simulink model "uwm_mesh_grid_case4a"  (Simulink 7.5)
settings: Solver=ode45  StartTime=0.0  StopTime=3.0  RelTol=1e-4
undefined symbols (not defined in the file or in its folder): D1, Delta, dfilt, DiscIntNeverNeededParam
libraries: powerlib x86, powerlib_extras x20, dsparch4 x6
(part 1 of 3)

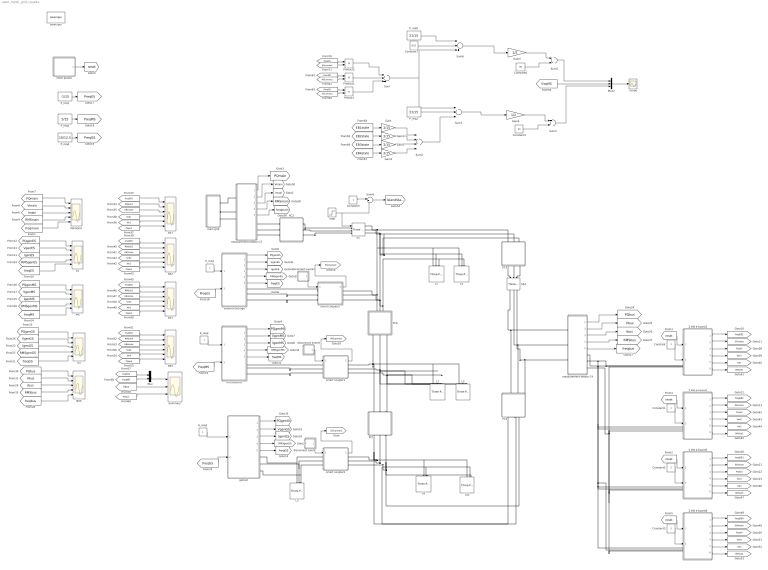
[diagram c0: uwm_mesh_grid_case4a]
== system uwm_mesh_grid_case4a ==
  2 kW e-board1 : Subsystem
  2 kW e-board2 : Subsystem
  2 kW e-board3 : Subsystem
  2 kW e-board4 : Subsystem
  BUS : Scope  NumInputPorts=5
  Constant{,1..3} (4 alike) : Constant  Value=2  OutDataType=fixdt(1, 16)  OutScaling=2^0
  Constant4 : Constant  Value=60  OutDataType=fixdt(1, 16)  OutScaling=2^0
  Constant5 : Constant  OutDataType=fixdt(1, 16)  OutScaling=2^0
  Constant6 : Constant  Value=60  OutDataType=fixdt(1, 16)  OutScaling=2^0
  Constant7 : Constant  Value=8/15  OutDataType=fixdt(1, 16)  OutScaling=2^0
  EB{1..4} (4 alike) : Scope  NumInputPorts=6
  ES : Scope  NumInputPorts=5
  E_req1 : Constant  OutDataType=fixdt(1, 16)  OutScaling=2^0
  E_req2 : Constant  OutDataType=fixdt(1, 16)  OutScaling=2^0
  E_req3 : Constant  OutDataType=fixdt(1, 16)  OutScaling=2^0
  GS : Scope  NumInputPorts=5
  Gain{,1..3} (4 alike) : Gain  Gain=2/15  ParameterDataType=fixdt(1, 16)  ParameterScaling=2^0  OutDataType=fixdt(1, 16)  OutScaling=2^0
  Gain4 : Gain  Gain=1/2  ParameterDataType=fixdt(1, 16)  ParameterScaling=2^0  OutDataType=fixdt(1, 16)  OutScaling=2^0
  Gain5 : Gain  Gain=1/2  ParameterDataType=fixdt(1, 16)  ParameterScaling=2^0  OutDataType=fixdt(1, 16)  OutScaling=2^0
  L{1..4,42} (5 alike) : powerlib/Elements/Three-Phase Series RLC Load  DialogController=POWERSYS.PowerSysDialog  PhysicalDomain=powersysdomain  SubClassName=unknown  LeftPortType=p1  RightPortType=p1  LConnTagsString=A|B|C  Configuration=Y (grounded)  NominalVoltage=208  NominalFrequency=60  ActivePower=4000  InductivePower=0  CapacitivePower=0  Measurements=None
  L5 : powerlib/Elements/Three-Phase Series RLC Load  DialogController=POWERSYS.PowerSysDialog  PhysicalDomain=powersysdomain  SubClassName=unknown  LeftPortType=p1  RightPortType=p1  LConnTagsString=A|B|C  Configuration=Y (grounded)  NominalVoltage=208  NominalFrequency=60  ActivePower=2000  InductivePower=0  CapacitivePower=0  Measurements=None
  L6 : powerlib/Elements/Three-Phase Series RLC Load  DialogController=POWERSYS.PowerSysDialog  PhysicalDomain=powersysdomain  SubClassName=unknown  LeftPortType=p1  RightPortType=p1  LConnTagsString=A|B|C  Configuration=Y (grounded)  NominalVoltage=208  NominalFrequency=60  ActivePower=2000  InductivePower=0  CapacitivePower=0  Measurements=None
  MS : Scope  NumInputPorts=5
  MainGrid : Scope  NumInputPorts=5
  Mux : Mux  Inputs=2
  Mux2 : Mux  Inputs=3
  PC2 : Subsystem  mask{R=.002810, L=.000679, C=2894.3}
  PC3 : Subsystem  mask{R=0.027352, L=.006600, C=288.6}
  PC4 : Subsystem  mask{R=.01688, L=.004070, C=336.7}
  PC5 : Subsystem  mask{R=.002600, L=.000640, C=2020.1}
  PC6 : Subsystem  mask{R=.013700, L=.003300, C=577.2}
  P_req1 : Constant  Value=-1/15  OutDataType=fixdt(1, 16)  OutScaling=2^0
  P_req2 : Constant  Value=21/15  OutDataType=fixdt(1, 16)  OutScaling=2^0
  P_req3 : Constant  Value=5/15  OutDataType=fixdt(1, 16)  OutScaling=2^0
  P_req4 : Constant  Value=10/12.5  OutDataType=fixdt(1, 16)  OutScaling=2^0
  P_req5 : Constant  Value=21/15  OutDataType=fixdt(1, 16)  OutScaling=2^0
  Product : Product  OutDataType=fixdt(1, 16)  OutScaling=2^0
  Product1 : Product  OutDataType=fixdt(1, 16)  OutScaling=2^0
  Product2 : Product  OutDataType=fixdt(1, 16)  OutScaling=2^0
  SS : powerlib/Elements/Three-Phase Breaker  DialogController=POWERSYS.PowerSysDialog  SystemSampleTime=-1  InitialState=closed  SwitchA=on  SwitchB=on  SwitchC=on  SwitchTimes=[1.]  External=on  BreakerResistance=.001  SnubberResistance=1e6  SnubberCapacitance=inf  Measurements=None
  SS3 : powerlib/Elements/Three-Phase Breaker  DialogController=POWERSYS.PowerSysDialog  SystemSampleTime=-1  InitialState=closed  SwitchA=on  SwitchB=on  SwitchC=on  SwitchTimes=[50]  External=off  BreakerResistance=.00001  SnubberResistance=1e10  SnubberCapacitance=inf  Measurements=None
  Scope : Scope
  Step : Step  Time=.5  Before=1  After=0  SampleTime=0
  Sum : Sum  Inputs=+++  OutDataType=fixdt(1, 16)  OutScaling=2^0
  Sum1 : Sum  Inputs=+--  OutDataType=fixdt(1, 16)  OutScaling=2^0
  Sum2 : Sum  Inputs=++++  OutDataType=fixdt(1, 16)  OutScaling=2^0
  Sum3 : Sum  OutDataType=fixdt(1, 16)  OutScaling=2^0
  Sum4 : Sum  Inputs=|+-  OutDataType=fixdt(1, 16)  OutScaling=2^0
  Sum5 : Sum  OutDataType=fixdt(1, 16)  OutScaling=2^0
  Sum6 : Sum  Inputs=--+  OutDataType=fixdt(1, 16)  OutScaling=2^0
  Summary : Scope  NumInputPorts=3
  disconnect event : Subsystem  mask{tstart=50, tstop=60}
      mask prompts: tstart "disconnect time"; tstop "connect time"
  disconnect event1 : Subsystem  mask{tstart=1, tstop=1.5}
      mask prompts: tstart "disconnect time"; tstop "connect time"
  disconnect event2 : Subsystem  mask{tstart=50, tstop=60}
      mask prompts: tstart "disconnect time"; tstop "connect time"
  external storage : Subsystem  AncestorBlock=|
      | UWM_blocks/inverter-based
      | DG (simplified)
      | 208V - 15kVA
  genset : Subsystem
  main grid : Subsystem
  measurement feeder C3 : Subsystem
  measurement feeder C4 : Subsystem
  microsource : Subsystem  AncestorBlock=|
      | UWM_blocks/inverter-based
      | DG (simplified)
      | 208V - 15kVA
  powergui : powerlib/powergui  Priority=1  SystemSampleTime=-1  SimulationMode=Discrete  SampleTime=20e-6  frequency=60  SPID=off  DisableSnubberDevices=off  DisableRonSwitches=off  DisableVfSwitches=off  SwTol=0  Interpol=off  frequencyindice=60  echomessages=off  HookPort=off  DisplayEquations=off  FunctionMessages=off  EnableUseOfTLC=off  x0status=steady  RestoreLinks=no  ResistiveCurrentMeasurement=off  Frange=[0:2:500]  Ylog=off  Xlog=on  ShowGrid=off  save=off  variable=ZData  ZoomFFT=on  StartTime=0.0  cycles=1  DisplayStyle=1  fundamental=60  FreqAxis=off  MaxFrequency=1000  frequencyindicesteady=1  RmsSteady=2  display=off  Ts=0  methode=off
  reset pulses : Subsystem  mask{tpulse=[50 100]}
  smart coupler1 : Subsystem
  smart coupler2 : Subsystem
  smart coupler3 : Subsystem
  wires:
  [PreqMS] -> microsource/2(P_req)
  E_req2/1 -> microsource/1(E_req)
  E_req1/1 -> external storage/1(E_req)
  E_req3/1 -> genset/1(Ereq)
  [PreqGS] -> genset/2(Preq)
  reset pulses/1(Out1) -> [reset]
  [reset] -> 2 kW e-board1/1(reset)
  2 kW e-board1/1(w) -> [freqEB1]
  2 kW e-board1/2(state) -> [EB1state]
  measurement feeder C3/3(I) -> [Imain]
  measurement feeder C3/1(PQ) -> [PQmain]
  [PreqES] -> external storage/2(P_req)
  P_req1/1 -> [PreqES]
  P_req3/1 -> [PreqMS]
  P_req4/1 -> [PreqGS]
  measurement feeder C3/2(V) -> [Vmain]
  [PQmain] -> MainGrid/1
  [Vmain] -> MainGrid/2
  [Imain] -> MainGrid/3
  [RMSmain] -> MainGrid/4
  external storage/5(freq) -> [freqES]
  external storage/3(I) -> [IgenES]
  external storage/2(V) -> [VgenES]
  external storage/1(PQ) -> [PQgenES]
  microsource/1(PQ) -> [PQgenMS]
  microsource/2(V) -> [VgenMS]
  microsource/3(I) -> [IgenMS]
  microsource/5(freq) -> [freqMS]
  genset/1(PQ) -> [PQgenGS]
  genset/2(V) -> [VgenGS]
  genset/3(I) -> [IgenGS]
  genset/5(freq) -> [freqGS]
  measurement feeder C4/1(PQ) -> [PQbus]
  measurement feeder C4/2(V) -> [Vbus]
  measurement feeder C4/3(I) -> [Ibus]
  measurement feeder C4/5(freq) -> [freqbus]
  measurement feeder C3/4(RMS) -> [RMSmain]
  external storage/4(RMS) -> [RMSgenES]
  microsource/4(RMS) -> [RMSgenMS]
  genset/4(RMS) -> [RMSgenGS]
  measurement feeder C3/5(freq) -> [freqmain]
  [freqmain] -> MainGrid/5
  [PQgenES] -> ES/1
  [VgenES] -> ES/2
  [IgenES] -> ES/3
  [RMSgenES] -> ES/4
  [freqES] -> ES/5
  [PQgenMS] -> MS/1
  [VgenMS] -> MS/2
  [IgenMS] -> MS/3
  [RMSgenMS] -> MS/4
  [freqMS] -> MS/5
  [PQgenGS] -> GS/1
  [VgenGS] -> GS/2
  [IgenGS] -> GS/3
  [RMSgenGS] -> GS/4
  [freqGS] -> GS/5
  measurement feeder C4/4(RMS) -> [RMSbus]
  [PQbus] -> BUS/1
  [Vbus] -> BUS/2
  [Ibus] -> BUS/3
  [RMSbus] -> BUS/4
  [freqbus] -> BUS/5
  Constant/1 -> 2 kW e-board1/2(priority)
  [freqEB1] -> EB1/1
  [RMSeb1] -> EB1/2
  [EB1state] -> EB1/3
  2 kW e-board1/3(PQ) -> [PQeb1]
  2 kW e-board1/4(V) -> [Veb1]
  2 kW e-board1/5(I) -> [Ieb1]
  2 kW e-board1/6(RMS) -> [RMSeb1]
  [PQeb1] -> EB1/6
  [Ieb1] -> EB1/5
  [Veb1] -> EB1/4
  [reset] -> 2 kW e-board2/1(reset)
  2 kW e-board2/1(w) -> [freqEB2]
  2 kW e-board2/2(state) -> [EB2state]
  Constant1/1 -> 2 kW e-board2/2(priority)
  2 kW e-board2/3(PQ) -> [PQeb2]
  2 kW e-board2/4(V) -> [Veb2]
  2 kW e-board2/5(I) -> [Ieb2]
  2 kW e-board2/6(RMS) -> [RMSeb2]
  [reset] -> 2 kW e-board3/1(reset)
  2 kW e-board3/1(w) -> [freqEB3]
  2 kW e-board3/2(state) -> [EB3state]
  Constant2/1 -> 2 kW e-board3/2(priority)
  2 kW e-board3/3(PQ) -> [PQeb3]
  2 kW e-board3/4(V) -> [Veb3]
  2 kW e-board3/5(I) -> [Ieb3]
  2 kW e-board3/6(RMS) -> [RMSeb3]
  [reset] -> 2 kW e-board4/1(reset)
  2 kW e-board4/1(w) -> [freqEB4]
  2 kW e-board4/2(state) -> [EB4state]
  Constant3/1 -> 2 kW e-board4/2(priority)
  2 kW e-board4/3(PQ) -> [PQeb4]
  2 kW e-board4/4(V) -> [Veb4]
  2 kW e-board4/5(I) -> [Ieb4]
  2 kW e-board4/6(RMS) -> [RMSeb4]
  [freqEB2] -> EB2/1
  [RMSeb2] -> EB2/2
  [EB2state] -> EB2/3
  [PQeb2] -> EB2/6
  [Ieb2] -> EB2/5
  [Veb2] -> EB2/4
  [freqEB3] -> EB3/1
  [RMSeb3] -> EB3/2
  [EB3state] -> EB3/3
  [PQeb3] -> EB3/6
  [Ieb3] -> EB3/5
  [Veb3] -> EB3/4
  [freqEB4] -> EB4/1
  [RMSeb4] -> EB4/2
  [EB4state] -> EB4/3
  [PQeb4] -> EB4/6
  [Ieb4] -> EB4/5
  [Veb4] -> EB4/4
  Step/1 -> SS/1, Sum4/2
  [freqEB4] -> Mux/1
  [freqMS] -> Mux/2
  [PQbus] -> Summary/3
  Mux/1 -> Summary/1
  [Vbus] -> Summary/2
  disconnect event/1(Out1) -> smart coupler2/1(event)
  Product2/1 -> Sum/1
  Product1/1 -> Sum/2
  smart coupler2/1(connected) -> [GSconnect]
  [PreqGS] -> Product/1
  [GSconnect] -> Product/2
  Product/1 -> Sum/3
  Constant5/1 -> Sum4/1
  Sum4/1 -> [IslandState]
  Constant6/1 -> Sum5/2
  Gain5/1 -> Sum5/1
  Sum6/1 -> Gain5/1
  [freqMS] -> Mux2/2
  Sum5/1 -> Mux2/1
  [EB1state] -> Gain/1
  P_req2/1 -> Sum1/2
  [EB2state] -> Gain1/1
  [EB3state] -> Gain2/1
  [EB4state] -> Gain3/1
  Gain1/1 -> Sum2/2
  Gain2/1 -> Sum2/3
  Gain/1 -> Sum2/1
  Gain3/1 -> Sum2/4
  Sum2/1 -> Sum1/3
  Constant4/1 -> Sum3/2
  Gain4/1 -> Sum3/1
  Sum1/1 -> Gain4/1
  Mux2/1 -> Scope/1
  Sum3/1 -> Mux2/3
  Sum/1 -> Sum1/1, Sum6/3
  Constant7/1 -> Sum6/2
  P_req5/1 -> Sum6/1
  disconnect event1/1(Out1) -> smart coupler1/1(event)
  smart coupler1/1(connected) -> [MSconnect]
  disconnect event2/1(Out1) -> smart coupler3/1(event)
  smart coupler3/1(connected) -> [ESconnect]
  [PreqMS] -> Product1/1
  [MSconnect] -> Product1/2
  [PreqES] -> Product2/1
  [ESconnect] -> Product2/2
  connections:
  measurement feeder C4/LConn1 -- PC4/RConn1 -- SS3/RConn1
  measurement feeder C4/LConn2 -- PC4/RConn2 -- SS3/RConn2
  measurement feeder C4/LConn3 -- PC4/RConn3 -- SS3/RConn3
  L42/LConn1 -- PC5/LConn1 -- PC4/LConn1 -- smart coupler2/RConn1 -- L6/LConn1
  L42/LConn3 -- PC4/LConn3 -- PC5/LConn3 -- smart coupler2/RConn3 -- L6/LConn3
  PC5/RConn1 -- L1/LConn1 -- L2/LConn1 -- PC6/LConn1 -- smart coupler1/RConn1
  L2/LConn2 -- L1/LConn2 -- PC5/RConn2 -- PC6/LConn2 -- smart coupler1/RConn2
  L2/LConn3 -- L1/LConn3 -- PC5/RConn3 -- PC6/LConn3 -- smart coupler1/RConn3
  main grid/RConn2 -- measurement feeder C3/LConn2
  main grid/RConn1 -- measurement feeder C3/LConn1
  measurement feeder C3/LConn3 -- main grid/RConn3
  measurement feeder C3/RConn1 -- PC2/LConn1
  measurement feeder C3/RConn2 -- PC2/LConn2
  measurement feeder C3/RConn3 -- PC2/LConn3
  PC2/RConn2 -- SS/LConn2
  PC2/RConn1 -- SS/LConn1
  SS/LConn3 -- PC2/RConn3
  SS3/LConn2 -- PC3/LConn2
  SS3/LConn3 -- PC3/LConn3
  SS3/LConn1 -- PC3/LConn1
  L5/LConn1 -- genset/RConn1 -- smart coupler2/LConn1
  L5/LConn2 -- genset/RConn2 -- smart coupler2/LConn2
  L5/LConn3 -- genset/RConn3 -- smart coupler2/LConn3
  measurement feeder C4/RConn2 -- 2 kW e-board1/LConn2 -- 2 kW e-board3/LConn2 -- 2 kW e-board4/LConn2 -- 2 kW e-board2/LConn2
  measurement feeder C4/RConn3 -- 2 kW e-board1/LConn3 -- 2 kW e-board2/LConn3 -- 2 kW e-board3/LConn3 -- 2 kW e-board4/LConn3
  2 kW e-board1/LConn1 -- 2 kW e-board3/LConn1 -- 2 kW e-board4/LConn1 -- 2 kW e-board2/LConn1 -- measurement feeder C4/RConn1
  PC6/RConn1 -- L3/LConn1 -- L4/LConn1 -- SS/RConn1 -- PC3/RConn1 -- smart coupler3/RConn1
  PC6/RConn2 -- L3/LConn2 -- L4/LConn2 -- SS/RConn2 -- PC3/RConn2 -- smart coupler3/RConn2
  PC6/RConn3 -- L3/LConn3 -- L4/LConn3 -- SS/RConn3 -- PC3/RConn3 -- smart coupler3/RConn3
  L42/LConn2 -- PC5/LConn2 -- smart coupler2/RConn2 -- PC4/LConn2 -- L6/LConn2
  microsource/RConn1 -- smart coupler1/LConn1
  smart coupler1/LConn2 -- microsource/RConn2
  smart coupler1/LConn3 -- microsource/RConn3
  smart coupler3/LConn1 -- external storage/RConn1
  smart coupler3/LConn2 -- external storage/RConn2
  smart coupler3/LConn3 -- external storage/RConn3

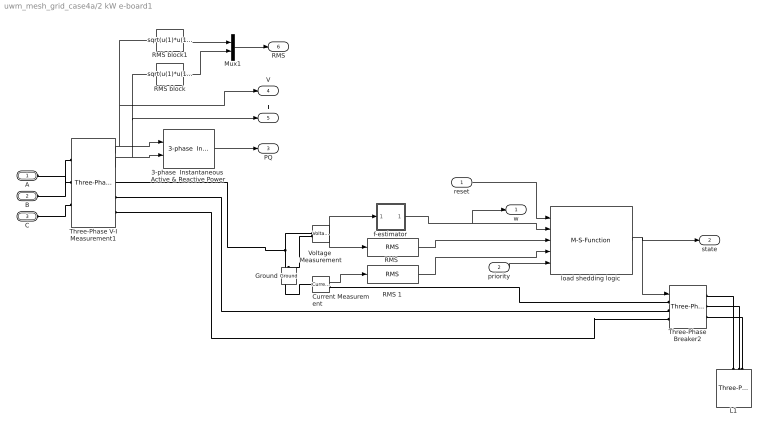
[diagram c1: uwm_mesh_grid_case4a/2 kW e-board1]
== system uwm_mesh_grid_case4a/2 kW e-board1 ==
  reset : Inport
  priority : Inport  Port=2
  3-phase  Instantaneous  Active & Reactive Power : powerlib_extras/Measurements/3-phase  Instantaneous  Active & Reactive Power  DialogController=POWERSYS.PowerSysDialog  SystemSampleTime=-1
  Current Measurement : powerlib/Measurements/Current Measurement  DialogController=POWERSYS.PowerSysDialog  SystemSampleTime=-1  PhasorSimulation=off  OutputType=Complex  PSBequivalent=0
  Ground : powerlib/Elements/Ground  DialogController=POWERSYS.PowerSysDialog  PhysicalDomain=powersysdomain  SubClassName=unknown  LeftPortType=p1  RightPortType=p1  LConnTagsString=a
  L1 : powerlib/Elements/Three-Phase Series RLC Load  DialogController=POWERSYS.PowerSysDialog  PhysicalDomain=powersysdomain  SubClassName=unknown  LeftPortType=p1  RightPortType=p1  LConnTagsString=A|B|C  Configuration=Y (grounded)  NominalVoltage=208  NominalFrequency=60  ActivePower=2000  InductivePower=0  CapacitivePower=0  Measurements=None
  Mux1 : Mux  Inputs=2
  "RMS " : powerlib_extras/Measurements/RMS  DialogController=POWERSYS.PowerSysDialog  SystemSampleTime=-1  f1=60
  RMS 1 : powerlib_extras/Measurements/RMS  DialogController=POWERSYS.PowerSysDialog  SystemSampleTime=-1  f1=60
  RMS block : Fcn  Expr=sqrt(u(1)*u(1)+u(2)*u(2)+u(3)*u(3))/sqrt(3)
  RMS block1 : Fcn  Expr=sqrt(u(1)*u(1)+u(2)*u(2)+u(3)*u(3))/sqrt(3)
  Three-Phase V-I Measurement1 : powerlib/Measurements/Three-Phase V-I Measurement  DialogController=POWERSYS.PowerSysDialog  SystemSampleTime=-1  VoltageMeasurement=phase-to-ground  SetLabelV=off  LabelV=Vabc  Vpu=off  VpuLL=off  CurrentMeasurement=yes  SetLabelI=off  LabelI=Iabc  Ipu=off  Pbase=100e6  Vbase=500e3  OutputType=Complex  PhasorSimulation=off  PSBequivalent=0
  Three-Phase Breaker2 : powerlib/Elements/Three-Phase Breaker  DialogController=POWERSYS.PowerSysDialog  SystemSampleTime=-1  InitialState=closed  SwitchA=on  SwitchB=on  SwitchC=on  SwitchTimes=[50]  External=on  BreakerResistance=0.001  SnubberResistance=1e6  SnubberCapacitance=inf  Measurements=None
  Voltage  Measurement : powerlib/Measurements/Voltage Measurement  DialogController=POWERSYS.PowerSysDialog  SystemSampleTime=-1  PhasorSimulation=off  OutputType=Complex  PSBequivalent=0
  f-estimator : Subsystem  mask{dt=0.010}
      mask prompts: dt "sample time"
  load shedding logic : M-S-Function  FunctionName=load_shedding_logic1
  A : PMIOPort  Port=1  Side=Left
  B : PMIOPort  Port=2  Side=Left
  C : PMIOPort  Port=3  Side=Left
  w : Outport  OutDataType=fixdt(1, 16)  OutScaling=2^0
  state : Outport  Port=2  OutDataType=fixdt(1, 16)  OutScaling=2^0
  PQ : Outport  Port=3  OutDataType=fixdt(1, 16)  OutScaling=2^0
  V : Outport  Port=4  OutDataType=fixdt(1, 16)  OutScaling=2^0
  I : Outport  Port=5  OutDataType=fixdt(1, 16)  OutScaling=2^0
  RMS : Outport  Port=6  OutDataType=fixdt(1, 16)  OutScaling=2^0
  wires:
  reset/1 -> load shedding logic/1
  Current Measurement/1 -> RMS 1/1
  Voltage  Measurement/1 -> "RMS "/1, f-estimator/1(v)
  f-estimator/1(w) -> load shedding logic/2, w/1
  "RMS "/1 -> load shedding logic/3
  RMS 1/1 -> load shedding logic/4
  load shedding logic/1 -> Three-Phase Breaker2/1, state/1
  priority/1 -> load shedding logic/5
  Three-Phase V-I Measurement1/1 -> 3-phase  Instantaneous  Active & Reactive Power/1, RMS block1/1, V/1
  Three-Phase V-I Measurement1/2 -> 3-phase  Instantaneous  Active & Reactive Power/2, RMS block/1, I/1
  3-phase  Instantaneous  Active & Reactive Power/1 -> PQ/1
  RMS block1/1 -> Mux1/1
  RMS block/1 -> Mux1/2
  Mux1/1 -> RMS/1
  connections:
  Voltage  Measurement/LConn1 -- Current Measurement/LConn1 -- Three-Phase V-I Measurement1/RConn1
  Voltage  Measurement/LConn2 -- Ground/LConn1
  Current Measurement/RConn1 -- Three-Phase Breaker2/LConn1
  L1/LConn1 -- Three-Phase Breaker2/RConn1
  L1/LConn2 -- Three-Phase Breaker2/RConn2
  L1/LConn3 -- Three-Phase Breaker2/RConn3
  Three-Phase V-I Measurement1/LConn1 -- A/RConn1
  Three-Phase V-I Measurement1/LConn2 -- B/RConn1
  Three-Phase V-I Measurement1/LConn3 -- C/RConn1
  Three-Phase V-I Measurement1/RConn2 -- Three-Phase Breaker2/LConn2
  Three-Phase V-I Measurement1/RConn3 -- Three-Phase Breaker2/LConn3

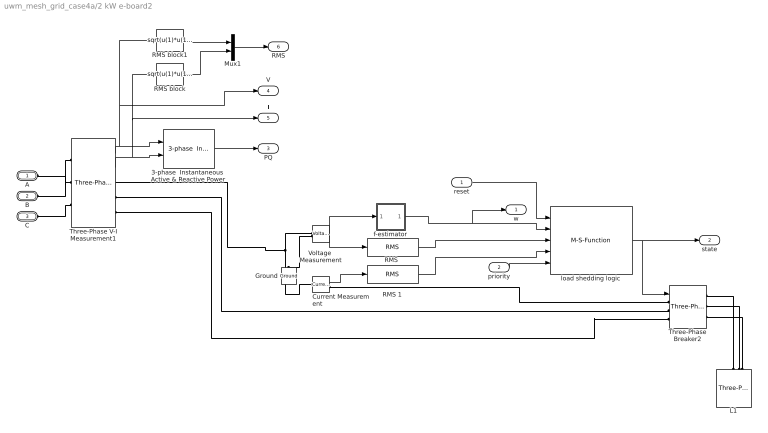
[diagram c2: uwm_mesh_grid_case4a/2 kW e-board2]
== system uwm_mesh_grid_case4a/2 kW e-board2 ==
  reset : Inport
  priority : Inport  Port=2
  3-phase  Instantaneous  Active & Reactive Power : powerlib_extras/Measurements/3-phase  Instantaneous  Active & Reactive Power  DialogController=POWERSYS.PowerSysDialog  SystemSampleTime=-1
  Current Measurement : powerlib/Measurements/Current Measurement  DialogController=POWERSYS.PowerSysDialog  SystemSampleTime=-1  PhasorSimulation=off  OutputType=Complex  PSBequivalent=0
  Ground : powerlib/Elements/Ground  DialogController=POWERSYS.PowerSysDialog  PhysicalDomain=powersysdomain  SubClassName=unknown  LeftPortType=p1  RightPortType=p1  LConnTagsString=a
  L1 : powerlib/Elements/Three-Phase Series RLC Load  DialogController=POWERSYS.PowerSysDialog  PhysicalDomain=powersysdomain  SubClassName=unknown  LeftPortType=p1  RightPortType=p1  LConnTagsString=A|B|C  Configuration=Y (grounded)  NominalVoltage=208  NominalFrequency=60  ActivePower=2000  InductivePower=0  CapacitivePower=0  Measurements=None
  Mux1 : Mux  Inputs=2
  "RMS " : powerlib_extras/Measurements/RMS  DialogController=POWERSYS.PowerSysDialog  SystemSampleTime=-1  f1=60
  RMS 1 : powerlib_extras/Measurements/RMS  DialogController=POWERSYS.PowerSysDialog  SystemSampleTime=-1  f1=60
  RMS block : Fcn  Expr=sqrt(u(1)*u(1)+u(2)*u(2)+u(3)*u(3))/sqrt(3)
  RMS block1 : Fcn  Expr=sqrt(u(1)*u(1)+u(2)*u(2)+u(3)*u(3))/sqrt(3)
  Three-Phase V-I Measurement1 : powerlib/Measurements/Three-Phase V-I Measurement  DialogController=POWERSYS.PowerSysDialog  SystemSampleTime=-1  VoltageMeasurement=phase-to-ground  SetLabelV=off  LabelV=Vabc  Vpu=off  VpuLL=off  CurrentMeasurement=yes  SetLabelI=off  LabelI=Iabc  Ipu=off  Pbase=100e6  Vbase=500e3  OutputType=Complex  PhasorSimulation=off  PSBequivalent=0
  Three-Phase Breaker2 : powerlib/Elements/Three-Phase Breaker  DialogController=POWERSYS.PowerSysDialog  SystemSampleTime=-1  InitialState=closed  SwitchA=on  SwitchB=on  SwitchC=on  SwitchTimes=[50]  External=on  BreakerResistance=0.001  SnubberResistance=1e6  SnubberCapacitance=inf  Measurements=None
  Voltage  Measurement : powerlib/Measurements/Voltage Measurement  DialogController=POWERSYS.PowerSysDialog  SystemSampleTime=-1  PhasorSimulation=off  OutputType=Complex  PSBequivalent=0
  f-estimator : Subsystem  mask{dt=0.010}
      mask prompts: dt "sample time"
  load shedding logic : M-S-Function  FunctionName=load_shedding_logic1
  A : PMIOPort  Port=1  Side=Left
  B : PMIOPort  Port=2  Side=Left
  C : PMIOPort  Port=3  Side=Left
  w : Outport  OutDataType=fixdt(1, 16)  OutScaling=2^0
  state : Outport  Port=2  OutDataType=fixdt(1, 16)  OutScaling=2^0
  PQ : Outport  Port=3  OutDataType=fixdt(1, 16)  OutScaling=2^0
  V : Outport  Port=4  OutDataType=fixdt(1, 16)  OutScaling=2^0
  I : Outport  Port=5  OutDataType=fixdt(1, 16)  OutScaling=2^0
  RMS : Outport  Port=6  OutDataType=fixdt(1, 16)  OutScaling=2^0
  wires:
  reset/1 -> load shedding logic/1
  Current Measurement/1 -> RMS 1/1
  Voltage  Measurement/1 -> "RMS "/1, f-estimator/1(v)
  f-estimator/1(w) -> load shedding logic/2, w/1
  "RMS "/1 -> load shedding logic/3
  RMS 1/1 -> load shedding logic/4
  load shedding logic/1 -> Three-Phase Breaker2/1, state/1
  priority/1 -> load shedding logic/5
  Three-Phase V-I Measurement1/1 -> 3-phase  Instantaneous  Active & Reactive Power/1, RMS block1/1, V/1
  Three-Phase V-I Measurement1/2 -> 3-phase  Instantaneous  Active & Reactive Power/2, RMS block/1, I/1
  3-phase  Instantaneous  Active & Reactive Power/1 -> PQ/1
  RMS block1/1 -> Mux1/1
  RMS block/1 -> Mux1/2
  Mux1/1 -> RMS/1
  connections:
  Voltage  Measurement/LConn1 -- Current Measurement/LConn1 -- Three-Phase V-I Measurement1/RConn1
  Voltage  Measurement/LConn2 -- Ground/LConn1
  Current Measurement/RConn1 -- Three-Phase Breaker2/LConn1
  L1/LConn1 -- Three-Phase Breaker2/RConn1
  L1/LConn2 -- Three-Phase Breaker2/RConn2
  L1/LConn3 -- Three-Phase Breaker2/RConn3
  Three-Phase V-I Measurement1/LConn1 -- A/RConn1
  Three-Phase V-I Measurement1/LConn2 -- B/RConn1
  Three-Phase V-I Measurement1/LConn3 -- C/RConn1
  Three-Phase V-I Measurement1/RConn2 -- Three-Phase Breaker2/LConn2
  Three-Phase V-I Measurement1/RConn3 -- Three-Phase Breaker2/LConn3

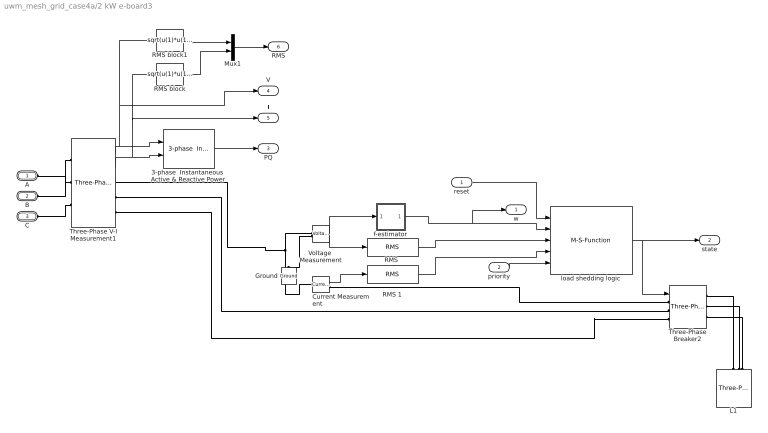
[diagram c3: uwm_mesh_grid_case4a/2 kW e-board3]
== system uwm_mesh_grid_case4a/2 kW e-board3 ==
  reset : Inport
  priority : Inport  Port=2
  3-phase  Instantaneous  Active & Reactive Power : powerlib_extras/Measurements/3-phase  Instantaneous  Active & Reactive Power  DialogController=POWERSYS.PowerSysDialog  SystemSampleTime=-1
  Current Measurement : powerlib/Measurements/Current Measurement  DialogController=POWERSYS.PowerSysDialog  SystemSampleTime=-1  PhasorSimulation=off  OutputType=Complex  PSBequivalent=0
  Ground : powerlib/Elements/Ground  DialogController=POWERSYS.PowerSysDialog  PhysicalDomain=powersysdomain  SubClassName=unknown  LeftPortType=p1  RightPortType=p1  LConnTagsString=a
  L1 : powerlib/Elements/Three-Phase Series RLC Load  DialogController=POWERSYS.PowerSysDialog  PhysicalDomain=powersysdomain  SubClassName=unknown  LeftPortType=p1  RightPortType=p1  LConnTagsString=A|B|C  Configuration=Y (grounded)  NominalVoltage=208  NominalFrequency=60  ActivePower=2000  InductivePower=0  CapacitivePower=0  Measurements=None
  Mux1 : Mux  Inputs=2
  "RMS " : powerlib_extras/Measurements/RMS  DialogController=POWERSYS.PowerSysDialog  SystemSampleTime=-1  f1=60
  RMS 1 : powerlib_extras/Measurements/RMS  DialogController=POWERSYS.PowerSysDialog  SystemSampleTime=-1  f1=60
  RMS block : Fcn  Expr=sqrt(u(1)*u(1)+u(2)*u(2)+u(3)*u(3))/sqrt(3)
  RMS block1 : Fcn  Expr=sqrt(u(1)*u(1)+u(2)*u(2)+u(3)*u(3))/sqrt(3)
  Three-Phase V-I Measurement1 : powerlib/Measurements/Three-Phase V-I Measurement  DialogController=POWERSYS.PowerSysDialog  SystemSampleTime=-1  VoltageMeasurement=phase-to-ground  SetLabelV=off  LabelV=Vabc  Vpu=off  VpuLL=off  CurrentMeasurement=yes  SetLabelI=off  LabelI=Iabc  Ipu=off  Pbase=100e6  Vbase=500e3  OutputType=Complex  PhasorSimulation=off  PSBequivalent=0
  Three-Phase Breaker2 : powerlib/Elements/Three-Phase Breaker  DialogController=POWERSYS.PowerSysDialog  SystemSampleTime=-1  InitialState=closed  SwitchA=on  SwitchB=on  SwitchC=on  SwitchTimes=[50]  External=on  BreakerResistance=0.001  SnubberResistance=1e6  SnubberCapacitance=inf  Measurements=None
  Voltage  Measurement : powerlib/Measurements/Voltage Measurement  DialogController=POWERSYS.PowerSysDialog  SystemSampleTime=-1  PhasorSimulation=off  OutputType=Complex  PSBequivalent=0
  f-estimator : Subsystem  mask{dt=0.010}
      mask prompts: dt "sample time"
  load shedding logic : M-S-Function  FunctionName=load_shedding_logic1
  A : PMIOPort  Port=1  Side=Left
  B : PMIOPort  Port=2  Side=Left
  C : PMIOPort  Port=3  Side=Left
  w : Outport  OutDataType=fixdt(1, 16)  OutScaling=2^0
  state : Outport  Port=2  OutDataType=fixdt(1, 16)  OutScaling=2^0
  PQ : Outport  Port=3  OutDataType=fixdt(1, 16)  OutScaling=2^0
  V : Outport  Port=4  OutDataType=fixdt(1, 16)  OutScaling=2^0
  I : Outport  Port=5  OutDataType=fixdt(1, 16)  OutScaling=2^0
  RMS : Outport  Port=6  OutDataType=fixdt(1, 16)  OutScaling=2^0
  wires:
  reset/1 -> load shedding logic/1
  Current Measurement/1 -> RMS 1/1
  Voltage  Measurement/1 -> "RMS "/1, f-estimator/1(v)
  f-estimator/1(w) -> load shedding logic/2, w/1
  "RMS "/1 -> load shedding logic/3
  RMS 1/1 -> load shedding logic/4
  load shedding logic/1 -> Three-Phase Breaker2/1, state/1
  priority/1 -> load shedding logic/5
  Three-Phase V-I Measurement1/1 -> 3-phase  Instantaneous  Active & Reactive Power/1, RMS block1/1, V/1
  Three-Phase V-I Measurement1/2 -> 3-phase  Instantaneous  Active & Reactive Power/2, RMS block/1, I/1
  3-phase  Instantaneous  Active & Reactive Power/1 -> PQ/1
  RMS block1/1 -> Mux1/1
  RMS block/1 -> Mux1/2
  Mux1/1 -> RMS/1
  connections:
  Voltage  Measurement/LConn1 -- Current Measurement/LConn1 -- Three-Phase V-I Measurement1/RConn1
  Voltage  Measurement/LConn2 -- Ground/LConn1
  Current Measurement/RConn1 -- Three-Phase Breaker2/LConn1
  L1/LConn1 -- Three-Phase Breaker2/RConn1
  L1/LConn2 -- Three-Phase Breaker2/RConn2
  L1/LConn3 -- Three-Phase Breaker2/RConn3
  Three-Phase V-I Measurement1/LConn1 -- A/RConn1
  Three-Phase V-I Measurement1/LConn2 -- B/RConn1
  Three-Phase V-I Measurement1/LConn3 -- C/RConn1
  Three-Phase V-I Measurement1/RConn2 -- Three-Phase Breaker2/LConn2
  Three-Phase V-I Measurement1/RConn3 -- Three-Phase Breaker2/LConn3

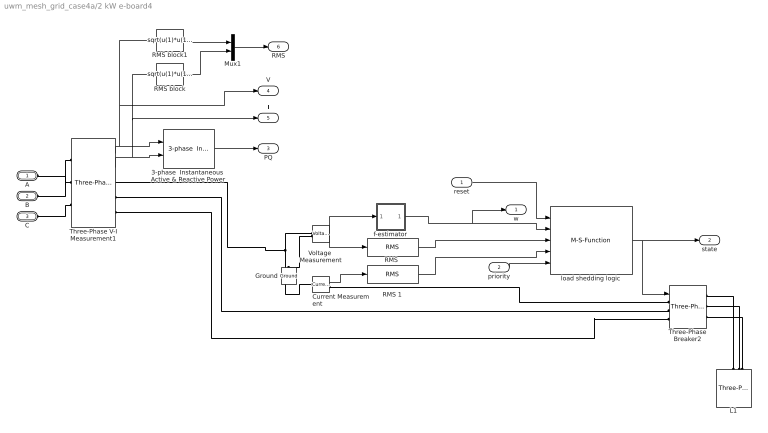
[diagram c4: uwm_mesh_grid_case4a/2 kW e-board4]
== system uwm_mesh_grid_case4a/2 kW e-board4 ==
  reset : Inport
  priority : Inport  Port=2
  3-phase  Instantaneous  Active & Reactive Power : powerlib_extras/Measurements/3-phase  Instantaneous  Active & Reactive Power  DialogController=POWERSYS.PowerSysDialog  SystemSampleTime=-1
  Current Measurement : powerlib/Measurements/Current Measurement  DialogController=POWERSYS.PowerSysDialog  SystemSampleTime=-1  PhasorSimulation=off  OutputType=Complex  PSBequivalent=0
  Ground : powerlib/Elements/Ground  DialogController=POWERSYS.PowerSysDialog  PhysicalDomain=powersysdomain  SubClassName=unknown  LeftPortType=p1  RightPortType=p1  LConnTagsString=a
  L1 : powerlib/Elements/Three-Phase Series RLC Load  DialogController=POWERSYS.PowerSysDialog  PhysicalDomain=powersysdomain  SubClassName=unknown  LeftPortType=p1  RightPortType=p1  LConnTagsString=A|B|C  Configuration=Y (grounded)  NominalVoltage=208  NominalFrequency=60  ActivePower=2000  InductivePower=0  CapacitivePower=0  Measurements=None
  Mux1 : Mux  Inputs=2
  "RMS " : powerlib_extras/Measurements/RMS  DialogController=POWERSYS.PowerSysDialog  SystemSampleTime=-1  f1=60
  RMS 1 : powerlib_extras/Measurements/RMS  DialogController=POWERSYS.PowerSysDialog  SystemSampleTime=-1  f1=60
  RMS block : Fcn  Expr=sqrt(u(1)*u(1)+u(2)*u(2)+u(3)*u(3))/sqrt(3)
  RMS block1 : Fcn  Expr=sqrt(u(1)*u(1)+u(2)*u(2)+u(3)*u(3))/sqrt(3)
  Three-Phase V-I Measurement1 : powerlib/Measurements/Three-Phase V-I Measurement  DialogController=POWERSYS.PowerSysDialog  SystemSampleTime=-1  VoltageMeasurement=phase-to-ground  SetLabelV=off  LabelV=Vabc  Vpu=off  VpuLL=off  CurrentMeasurement=yes  SetLabelI=off  LabelI=Iabc  Ipu=off  Pbase=100e6  Vbase=500e3  OutputType=Complex  PhasorSimulation=off  PSBequivalent=0
  Three-Phase Breaker2 : powerlib/Elements/Three-Phase Breaker  DialogController=POWERSYS.PowerSysDialog  SystemSampleTime=-1  InitialState=closed  SwitchA=on  SwitchB=on  SwitchC=on  SwitchTimes=[50]  External=on  BreakerResistance=0.001  SnubberResistance=1e6  SnubberCapacitance=inf  Measurements=None
  Voltage  Measurement : powerlib/Measurements/Voltage Measurement  DialogController=POWERSYS.PowerSysDialog  SystemSampleTime=-1  PhasorSimulation=off  OutputType=Complex  PSBequivalent=0
  f-estimator : Subsystem  mask{dt=0.010}
      mask prompts: dt "sample time"
  load shedding logic : M-S-Function  FunctionName=load_shedding_logic1
  A : PMIOPort  Port=1  Side=Left
  B : PMIOPort  Port=2  Side=Left
  C : PMIOPort  Port=3  Side=Left
  w : Outport  OutDataType=fixdt(1, 16)  OutScaling=2^0
  state : Outport  Port=2  OutDataType=fixdt(1, 16)  OutScaling=2^0
  PQ : Outport  Port=3  OutDataType=fixdt(1, 16)  OutScaling=2^0
  V : Outport  Port=4  OutDataType=fixdt(1, 16)  OutScaling=2^0
  I : Outport  Port=5  OutDataType=fixdt(1, 16)  OutScaling=2^0
  RMS : Outport  Port=6  OutDataType=fixdt(1, 16)  OutScaling=2^0
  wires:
  reset/1 -> load shedding logic/1
  Current Measurement/1 -> RMS 1/1
  Voltage  Measurement/1 -> "RMS "/1, f-estimator/1(v)
  f-estimator/1(w) -> load shedding logic/2, w/1
  "RMS "/1 -> load shedding logic/3
  RMS 1/1 -> load shedding logic/4
  load shedding logic/1 -> Three-Phase Breaker2/1, state/1
  priority/1 -> load shedding logic/5
  Three-Phase V-I Measurement1/1 -> 3-phase  Instantaneous  Active & Reactive Power/1, RMS block1/1, V/1
  Three-Phase V-I Measurement1/2 -> 3-phase  Instantaneous  Active & Reactive Power/2, RMS block/1, I/1
  3-phase  Instantaneous  Active & Reactive Power/1 -> PQ/1
  RMS block1/1 -> Mux1/1
  RMS block/1 -> Mux1/2
  Mux1/1 -> RMS/1
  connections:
  Voltage  Measurement/LConn1 -- Current Measurement/LConn1 -- Three-Phase V-I Measurement1/RConn1
  Voltage  Measurement/LConn2 -- Ground/LConn1
  Current Measurement/RConn1 -- Three-Phase Breaker2/LConn1
  L1/LConn1 -- Three-Phase Breaker2/RConn1
  L1/LConn2 -- Three-Phase Breaker2/RConn2
  L1/LConn3 -- Three-Phase Breaker2/RConn3
  Three-Phase V-I Measurement1/LConn1 -- A/RConn1
  Three-Phase V-I Measurement1/LConn2 -- B/RConn1
  Three-Phase V-I Measurement1/LConn3 -- C/RConn1
  Three-Phase V-I Measurement1/RConn2 -- Three-Phase Breaker2/LConn2
  Three-Phase V-I Measurement1/RConn3 -- Three-Phase Breaker2/LConn3

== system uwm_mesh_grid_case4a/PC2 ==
  Ground : powerlib/Elements/Ground  DialogController=POWERSYS.PowerSysDialog  PhysicalDomain=powersysdomain  SubClassName=unknown  LeftPortType=p1  RightPortType=p1  LConnTagsString=a
  Three-Phase Parallel RLC Branch : powerlib/Elements/Three-Phase Parallel RLC Branch  DialogController=POWERSYS.PowerSysDialog  PhysicalDomain=powersysdomain  SubClassName=unknown  LeftPortType=p1  RightPortType=p1  LConnTagsString=A|B|C  RConnTagsString=A|B|C  BranchType=C  Resistance=1  Inductance=1e-3  Capacitance=1/(C*2*pi*60)  Measurements=None
  Three-Phase Series RLC Branch3 : powerlib/Elements/Three-Phase Series RLC Branch  DialogController=POWERSYS.PowerSysDialog  PhysicalDomain=powersysdomain  SubClassName=unknown  LeftPortType=p1  RightPortType=p1  LConnTagsString=A|B|C  RConnTagsString=A|B|C  BranchType=RL  Resistance=R  Inductance=L/(2*pi*60)  Capacitance=1/(336*2*pi*60)  Measurements=None
  A* : PMIOPort  Tag=PMCPort  Port=1  Side=Right
  B* : PMIOPort  Tag=PMCPort  Port=2  Side=Right
  C* : PMIOPort  Tag=PMCPort  Port=3  Side=Right
  A : PMIOPort  Tag=PMCPort  Port=4  Side=Left
  B : PMIOPort  Tag=PMCPort  Port=5  Side=Left
  C : PMIOPort  Tag=PMCPort  Port=6  Side=Left
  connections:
  Three-Phase Parallel RLC Branch/LConn1 -- A*/RConn1 -- Three-Phase Series RLC Branch3/LConn1
  Three-Phase Parallel RLC Branch/LConn2 -- B*/RConn1 -- Three-Phase Series RLC Branch3/LConn2
  Three-Phase Parallel RLC Branch/LConn3 -- C*/RConn1 -- Three-Phase Series RLC Branch3/LConn3
  Three-Phase Series RLC Branch3/RConn1 -- A/RConn1
  Three-Phase Series RLC Branch3/RConn2 -- B/RConn1
  Three-Phase Series RLC Branch3/RConn3 -- C/RConn1
  Ground/LConn1 -- Three-Phase Parallel RLC Branch/RConn2 -- Three-Phase Parallel RLC Branch/RConn3 -- Three-Phase Parallel RLC Branch/RConn1

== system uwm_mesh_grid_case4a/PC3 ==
  Ground : powerlib/Elements/Ground  DialogController=POWERSYS.PowerSysDialog  PhysicalDomain=powersysdomain  SubClassName=unknown  LeftPortType=p1  RightPortType=p1  LConnTagsString=a
  Three-Phase Parallel RLC Branch : powerlib/Elements/Three-Phase Parallel RLC Branch  DialogController=POWERSYS.PowerSysDialog  PhysicalDomain=powersysdomain  SubClassName=unknown  LeftPortType=p1  RightPortType=p1  LConnTagsString=A|B|C  RConnTagsString=A|B|C  BranchType=C  Resistance=1  Inductance=1e-3  Capacitance=1/(C*2*pi*60)  Measurements=None
  Three-Phase Series RLC Branch3 : powerlib/Elements/Three-Phase Series RLC Branch  DialogController=POWERSYS.PowerSysDialog  PhysicalDomain=powersysdomain  SubClassName=unknown  LeftPortType=p1  RightPortType=p1  LConnTagsString=A|B|C  RConnTagsString=A|B|C  BranchType=RL  Resistance=R  Inductance=L/(2*pi*60)  Capacitance=1/(336*2*pi*60)  Measurements=None
  A* : PMIOPort  Tag=PMCPort  Port=1  Side=Right
  B* : PMIOPort  Tag=PMCPort  Port=2  Side=Right
  C* : PMIOPort  Tag=PMCPort  Port=3  Side=Right
  A : PMIOPort  Tag=PMCPort  Port=4  Side=Left
  B : PMIOPort  Tag=PMCPort  Port=5  Side=Left
  C : PMIOPort  Tag=PMCPort  Port=6  Side=Left
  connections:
  Three-Phase Parallel RLC Branch/LConn1 -- A*/RConn1 -- Three-Phase Series RLC Branch3/LConn1
  Three-Phase Parallel RLC Branch/LConn2 -- B*/RConn1 -- Three-Phase Series RLC Branch3/LConn2
  Three-Phase Parallel RLC Branch/LConn3 -- C*/RConn1 -- Three-Phase Series RLC Branch3/LConn3
  Three-Phase Series RLC Branch3/RConn1 -- A/RConn1
  Three-Phase Series RLC Branch3/RConn2 -- B/RConn1
  Three-Phase Series RLC Branch3/RConn3 -- C/RConn1
  Ground/LConn1 -- Three-Phase Parallel RLC Branch/RConn2 -- Three-Phase Parallel RLC Branch/RConn1 -- Three-Phase Parallel RLC Branch/RConn3

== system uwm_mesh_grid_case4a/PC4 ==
  Ground : powerlib/Elements/Ground  DialogController=POWERSYS.PowerSysDialog  PhysicalDomain=powersysdomain  SubClassName=unknown  LeftPortType=p1  RightPortType=p1  LConnTagsString=a
  Three-Phase Parallel RLC Branch : powerlib/Elements/Three-Phase Parallel RLC Branch  DialogController=POWERSYS.PowerSysDialog  PhysicalDomain=powersysdomain  SubClassName=unknown  LeftPortType=p1  RightPortType=p1  LConnTagsString=A|B|C  RConnTagsString=A|B|C  BranchType=C  Resistance=1  Inductance=1e-3  Capacitance=1/(C*2*pi*60)  Measurements=None
  Three-Phase Series RLC Branch3 : powerlib/Elements/Three-Phase Series RLC Branch  DialogController=POWERSYS.PowerSysDialog  PhysicalDomain=powersysdomain  SubClassName=unknown  LeftPortType=p1  RightPortType=p1  LConnTagsString=A|B|C  RConnTagsString=A|B|C  BranchType=RL  Resistance=R  Inductance=L/(2*pi*60)  Capacitance=1/(336*2*pi*60)  Measurements=None
  A* : PMIOPort  Tag=PMCPort  Port=1  Side=Right
  B* : PMIOPort  Tag=PMCPort  Port=2  Side=Right
  C* : PMIOPort  Tag=PMCPort  Port=3  Side=Right
  A : PMIOPort  Tag=PMCPort  Port=4  Side=Left
  B : PMIOPort  Tag=PMCPort  Port=5  Side=Left
  C : PMIOPort  Tag=PMCPort  Port=6  Side=Left
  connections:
  A*/RConn1 -- Three-Phase Series RLC Branch3/LConn1 -- Three-Phase Parallel RLC Branch/LConn1
  B*/RConn1 -- Three-Phase Series RLC Branch3/LConn2 -- Three-Phase Parallel RLC Branch/LConn2
  C*/RConn1 -- Three-Phase Series RLC Branch3/LConn3 -- Three-Phase Parallel RLC Branch/LConn3
  Three-Phase Series RLC Branch3/RConn1 -- A/RConn1
  Three-Phase Series RLC Branch3/RConn2 -- B/RConn1
  Three-Phase Series RLC Branch3/RConn3 -- C/RConn1
  Ground/LConn1 -- Three-Phase Parallel RLC Branch/RConn2 -- Three-Phase Parallel RLC Branch/RConn3 -- Three-Phase Parallel RLC Branch/RConn1

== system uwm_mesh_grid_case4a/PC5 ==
  Ground : powerlib/Elements/Ground  DialogController=POWERSYS.PowerSysDialog  PhysicalDomain=powersysdomain  SubClassName=unknown  LeftPortType=p1  RightPortType=p1  LConnTagsString=a
  Three-Phase Parallel RLC Branch : powerlib/Elements/Three-Phase Parallel RLC Branch  DialogController=POWERSYS.PowerSysDialog  PhysicalDomain=powersysdomain  SubClassName=unknown  LeftPortType=p1  RightPortType=p1  LConnTagsString=A|B|C  RConnTagsString=A|B|C  BranchType=C  Resistance=1  Inductance=1e-3  Capacitance=1/(C*2*pi*60)  Measurements=None
  Three-Phase Series RLC Branch3 : powerlib/Elements/Three-Phase Series RLC Branch  DialogController=POWERSYS.PowerSysDialog  PhysicalDomain=powersysdomain  SubClassName=unknown  LeftPortType=p1  RightPortType=p1  LConnTagsString=A|B|C  RConnTagsString=A|B|C  BranchType=RL  Resistance=R  Inductance=L/(2*pi*60)  Capacitance=1/(336*2*pi*60)  Measurements=None
  A* : PMIOPort  Tag=PMCPort  Port=1  Side=Right
  B* : PMIOPort  Tag=PMCPort  Port=2  Side=Right
  C* : PMIOPort  Tag=PMCPort  Port=3  Side=Right
  A : PMIOPort  Tag=PMCPort  Port=4  Side=Left
  B : PMIOPort  Tag=PMCPort  Port=5  Side=Left
  C : PMIOPort  Tag=PMCPort  Port=6  Side=Left
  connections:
  Three-Phase Parallel RLC Branch/LConn1 -- A*/RConn1 -- Three-Phase Series RLC Branch3/LConn1
  Three-Phase Parallel RLC Branch/LConn2 -- B*/RConn1 -- Three-Phase Series RLC Branch3/LConn2
  Three-Phase Parallel RLC Branch/LConn3 -- C*/RConn1 -- Three-Phase Series RLC Branch3/LConn3
  Three-Phase Series RLC Branch3/RConn1 -- A/RConn1
  Three-Phase Series RLC Branch3/RConn2 -- B/RConn1
  Three-Phase Series RLC Branch3/RConn3 -- C/RConn1
  Ground/LConn1 -- Three-Phase Parallel RLC Branch/RConn2 -- Three-Phase Parallel RLC Branch/RConn3 -- Three-Phase Parallel RLC Branch/RConn1

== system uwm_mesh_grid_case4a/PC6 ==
  Ground : powerlib/Elements/Ground  DialogController=POWERSYS.PowerSysDialog  PhysicalDomain=powersysdomain  SubClassName=unknown  LeftPortType=p1  RightPortType=p1  LConnTagsString=a
  Three-Phase Parallel RLC Branch : powerlib/Elements/Three-Phase Parallel RLC Branch  DialogController=POWERSYS.PowerSysDialog  PhysicalDomain=powersysdomain  SubClassName=unknown  LeftPortType=p1  RightPortType=p1  LConnTagsString=A|B|C  RConnTagsString=A|B|C  BranchType=C  Resistance=1  Inductance=1e-3  Capacitance=1/(C*2*pi*60)  Measurements=None
  Three-Phase Series RLC Branch3 : powerlib/Elements/Three-Phase Series RLC Branch  DialogController=POWERSYS.PowerSysDialog  PhysicalDomain=powersysdomain  SubClassName=unknown  LeftPortType=p1  RightPortType=p1  LConnTagsString=A|B|C  RConnTagsString=A|B|C  BranchType=RL  Resistance=R  Inductance=L/(2*pi*60)  Capacitance=1/(336*2*pi*60)  Measurements=None
  A* : PMIOPort  Tag=PMCPort  Port=1  Side=Right
  B* : PMIOPort  Tag=PMCPort  Port=2  Side=Right
  C* : PMIOPort  Tag=PMCPort  Port=3  Side=Right
  A : PMIOPort  Tag=PMCPort  Port=4  Side=Left
  B : PMIOPort  Tag=PMCPort  Port=5  Side=Left
  C : PMIOPort  Tag=PMCPort  Port=6  Side=Left
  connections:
  Three-Phase Parallel RLC Branch/LConn1 -- A*/RConn1 -- Three-Phase Series RLC Branch3/LConn1
  Three-Phase Parallel RLC Branch/LConn2 -- B*/RConn1 -- Three-Phase Series RLC Branch3/LConn2
  Three-Phase Parallel RLC Branch/LConn3 -- C*/RConn1 -- Three-Phase Series RLC Branch3/LConn3
  Three-Phase Series RLC Branch3/RConn1 -- A/RConn1
  Three-Phase Series RLC Branch3/RConn2 -- B/RConn1
  Three-Phase Series RLC Branch3/RConn3 -- C/RConn1
  Ground/LConn1 -- Three-Phase Parallel RLC Branch/RConn2 -- Three-Phase Parallel RLC Branch/RConn3 -- Three-Phase Parallel RLC Branch/RConn1

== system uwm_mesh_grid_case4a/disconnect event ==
  Step1 : Step  Time=[tstart]  Before=1  After=0  SampleTime=0
  Step2 : Step  Time=[tstop]  SampleTime=0
  Sum : Sum  OutDataType=fixdt(1, 16)  OutScaling=2^0
  Out1 : Outport
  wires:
  Step2/1 -> Sum/2
  Step1/1 -> Sum/1
  Sum/1 -> Out1/1

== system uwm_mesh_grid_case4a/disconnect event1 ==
  Step1 : Step  Time=[tstart]  Before=1  After=0  SampleTime=0
  Step2 : Step  Time=[tstop]  SampleTime=0
  Sum : Sum  OutDataType=fixdt(1, 16)  OutScaling=2^0
  Out1 : Outport
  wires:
  Step2/1 -> Sum/2
  Step1/1 -> Sum/1
  Sum/1 -> Out1/1

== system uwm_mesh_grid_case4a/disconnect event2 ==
  Step1 : Step  Time=[tstart]  Before=1  After=0  SampleTime=0
  Step2 : Step  Time=[tstop]  SampleTime=0
  Sum : Sum  OutDataType=fixdt(1, 16)  OutScaling=2^0
  Out1 : Outport
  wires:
  Step2/1 -> Sum/2
  Step1/1 -> Sum/1
  Sum/1 -> Out1/1

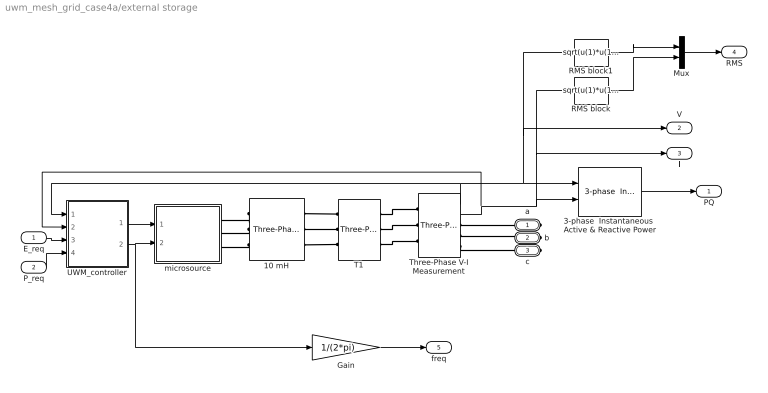
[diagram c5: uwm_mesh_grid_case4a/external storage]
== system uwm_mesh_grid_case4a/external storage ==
  E_req : Inport
  P_req : Inport  Port=2
  10 mH : powerlib/Elements/Three-Phase Series RLC Branch  DialogController=POWERSYS.PowerSysDialog  PhysicalDomain=powersysdomain  SubClassName=unknown  LeftPortType=p1  RightPortType=p1  LConnTagsString=A|B|C  RConnTagsString=A|B|C  BranchType=L  Resistance=.0028  Inductance=5e-3  Capacitance=1e-6  Measurements=None
  3-phase  Instantaneous  Active & Reactive Power : powerlib_extras/Measurements/3-phase  Instantaneous  Active & Reactive Power  DialogController=POWERSYS.PowerSysDialog  SystemSampleTime=-1
  Gain : Gain  Gain=1/(2*pi)  ParameterDataType=fixdt(1, 16)  ParameterScaling=2^0  OutDataType=fixdt(1, 16)  OutScaling=2^0
  Mux : Mux  Inputs=2
  RMS block : Fcn  Expr=sqrt(u(1)*u(1)+u(2)*u(2)+u(3)*u(3))/sqrt(3)
  RMS block1 : Fcn  Expr=sqrt(u(1)*u(1)+u(2)*u(2)+u(3)*u(3))/sqrt(3)
  T1 : powerlib/Elements/Three-Phase Transformer (Two Windings)  DialogController=POWERSYS.PowerSysDialog  SystemSampleTime=-1  Winding1Connection=Delta (D1)  UNITS=SI  NominalPower=[ 45e3 , 60 ]  Winding1=[208 0.02688 0.1075/(2*pi*60)]  Winding2Connection=Yg  Winding2=[208 0.005047 .0201/(2*pi*60)]  SetSaturation=off  Rm=100.e6  Lm=7650.8  Saturation=[0 0;1359.8 0.93633;5.6659e+05 1.186]  Hysteresis=off  DataFile='hysteresis'  SetInitialFlux=off  InitialFluxes=[0.62422 -0.62422 0.54618]  Measurements=None  MoreParameters=off  BreakLoop=off  DataType=on  TransfoNumber=1
  Three-Phase V-I Measurement : powerlib/Measurements/Three-Phase V-I Measurement  DialogController=POWERSYS.PowerSysDialog  SystemSampleTime=-1  VoltageMeasurement=phase-to-ground  SetLabelV=off  LabelV=Vabc  Vpu=off  VpuLL=off  CurrentMeasurement=yes  SetLabelI=off  LabelI=Iabc  Ipu=off  Pbase=100e6  Vbase=500e3  OutputType=Complex  PhasorSimulation=off  PSBequivalent=0
  UWM_controller : Subsystem  mask{Vbase=208, Sbase=15000}
  microsource : Subsystem
  a : PMIOPort  Port=1  Side=Right
  b : PMIOPort  Port=2  Side=Right
  c : PMIOPort  Port=3  Side=Right
  PQ : Outport  OutDataType=fixdt(1, 16)  OutScaling=2^0
  V : Outport  Port=2  OutDataType=fixdt(1, 16)  OutScaling=2^0
  I : Outport  Port=3  OutDataType=fixdt(1, 16)  OutScaling=2^0
  RMS : Outport  Port=4  OutDataType=fixdt(1, 16)  OutScaling=2^0
  freq : Outport  Port=5  OutDataType=fixdt(1, 16)  OutScaling=2^0
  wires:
  E_req/1 -> UWM_controller/3(E_req)
  P_req/1 -> UWM_controller/4(P_req)
  Three-Phase V-I Measurement/1 -> UWM_controller/1(v_meas), 3-phase  Instantaneous  Active & Reactive Power/1, RMS block1/1, V/1
  Three-Phase V-I Measurement/2 -> UWM_controller/2(i_meas), 3-phase  Instantaneous  Active & Reactive Power/2, RMS block/1, I/1
  UWM_controller/1(Vpk) -> microsource/1(Vpk)
  UWM_controller/2(w) -> microsource/2(w), Gain/1
  Gain/1 -> freq/1
  3-phase  Instantaneous  Active & Reactive Power/1 -> PQ/1
  RMS block1/1 -> Mux/1
  RMS block/1 -> Mux/2
  Mux/1 -> RMS/1
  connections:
  b/RConn1 -- Three-Phase V-I Measurement/RConn2
  Three-Phase V-I Measurement/RConn3 -- c/RConn1
  10 mH/LConn2 -- microsource/RConn2
  10 mH/LConn1 -- microsource/RConn1
  10 mH/LConn3 -- microsource/RConn3
  T1/LConn1 -- 10 mH/RConn1
  T1/LConn2 -- 10 mH/RConn2
  T1/LConn3 -- 10 mH/RConn3
  T1/RConn1 -- Three-Phase V-I Measurement/LConn1
  T1/RConn2 -- Three-Phase V-I Measurement/LConn2
  T1/RConn3 -- Three-Phase V-I Measurement/LConn3
  a/RConn1 -- Three-Phase V-I Measurement/RConn1

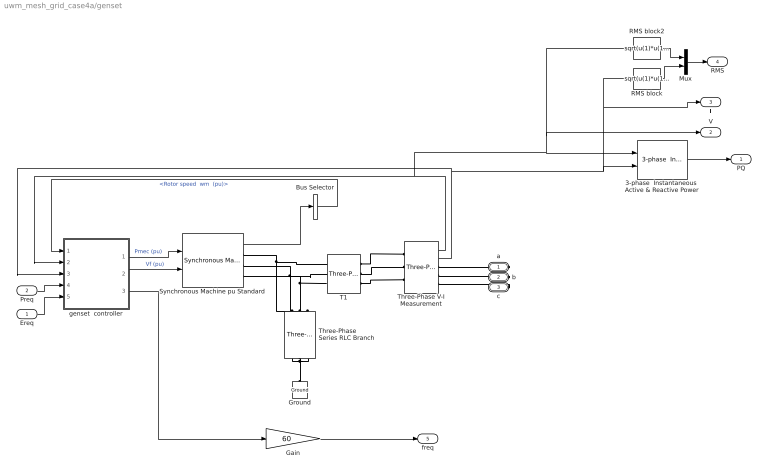
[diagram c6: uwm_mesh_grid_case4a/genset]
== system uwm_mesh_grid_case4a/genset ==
  Ereq : Inport  OutDataType=fixdt(1, 16)  OutScaling=2^0
  Preq : Inport  Port=2  OutDataType=fixdt(1, 16)  OutScaling=2^0
  3-phase  Instantaneous  Active & Reactive Power : powerlib_extras/Measurements/3-phase  Instantaneous  Active & Reactive Power  DialogController=POWERSYS.PowerSysDialog  SystemSampleTime=-1
  Bus Selector : BusSelector  OutputSignals="Mechanical.Rotor speed  wm  (pu)"
  Gain : Gain  Gain=60  ParameterDataType=fixdt(1, 16)  ParameterScaling=2^0  OutDataType=fixdt(1, 16)  OutScaling=2^0
  Ground : powerlib/Elements/Ground  DialogController=POWERSYS.PowerSysDialog  PhysicalDomain=powersysdomain  SubClassName=unknown  LeftPortType=p1  RightPortType=p1  LConnTagsString=a
  Mux : Mux  Inputs=2
  RMS block : Fcn  Expr=sqrt(u(1)*u(1)+u(2)*u(2)+u(3)*u(3))/sqrt(3)
  RMS block2 : Fcn  Expr=sqrt(u(1)*u(1)+u(2)*u(2)+u(3)*u(3))/sqrt(3)
  Synchronous Machine pu Standard : powerlib/Machines/Synchronous Machine pu Standard  DialogController=POWERSYS.PowerSysDialog  SystemSampleTime=-1  PresetModel=No  MechanicalLoad=Mechanical power Pm  ShowDetailedParameters=on  RotorType=Salient-pole  NominalParameters="[ 12500  208   60]"  Reactances1=[ 1.81, 0.3, 0.23, 1.76, 0.65, 0.25, 0.15 ]  Reactances2="[ 1.204, 0.125, 0.056, 0.533,  0.051,  0.037 ]"  dAxisTimeConstants=Short-circuit  qAxisTimeConstants=Short-circuit  TimeConstants1="[ 4.4849  0.0681  0.1  ]"  TimeConstants2=[ 8.0, 0.03, 1.0, 0.07 ]  TimeConstants3="[  .35523  0.00015  0.067  ]"  TimeConstants4=[ 8.0, 0.03, 0.3371, 0.0295 ]  TimeConstants5=[ 1.01, 0.053, 0.1 ]  TimeConstants6=[ 1.3201, 0.023, 1.0, 0.07 ]  TimeConstants7=[0.35523 0.00015 0.0067]  TimeConstants8=[ 1.3201, 0.0231, 0.3371, 0.0295 ]  StatorResistance=0.0217  Mechanical=[ .19 0 2 ]  PolePairs=2  InitialConditions="[ 0  0  0  0  0  0  0  0  1 ]"  SetSaturation=off  Saturation=[0.6404,0.7127,0.8441,0.9214,0.9956,1.082,1.19,1.316,1.457;0.7,0.7698,0.8872,0.9466,0.9969,1.046,1.1,1.151,1.201]  Units=per unit standard parameters  LoadFlowParameters=[1 0 0 0 0]  TsPowergui=0  TsBlock=-1  IterativeModel=Forward Euler
  T1 : powerlib/Elements/Three-Phase Transformer (Two Windings)  DialogController=POWERSYS.PowerSysDialog  SystemSampleTime=-1  Winding1Connection=Delta (D1)  UNITS=SI  NominalPower=[ 45e3 , 60 ]  Winding1=[208 .02688 .10752/(2*pi*60)]  Winding2Connection=Yg  Winding2=[208 .005047 .201899/(2*pi*60)]  SetSaturation=off  Rm=1e+08  Lm=7650.8  Saturation=[0 0;1359.8 0.93633;5.6659e+05 1.186]  Hysteresis=off  DataFile='hysteresis'  SetInitialFlux=off  InitialFluxes=[0.62422 -0.62422 0.54618]  Measurements=None  MoreParameters=off  BreakLoop=off  DataType=on  TransfoNumber=1
  Three-Phase Series RLC Branch : powerlib/Elements/Three-Phase Series RLC Branch  DialogController=POWERSYS.PowerSysDialog  PhysicalDomain=powersysdomain  SubClassName=unknown  LeftPortType=p1  RightPortType=p1  LConnTagsString=A|B|C  RConnTagsString=A|B|C  BranchType=C  Resistance=1  Inductance=1e-3  Capacitance=1.e-4  Measurements=None
  Three-Phase V-I Measurement : powerlib/Measurements/Three-Phase V-I Measurement  DialogController=POWERSYS.PowerSysDialog  SystemSampleTime=-1  VoltageMeasurement=phase-to-ground  SetLabelV=off  LabelV=Vabc  Vpu=off  VpuLL=off  CurrentMeasurement=yes  SetLabelI=off  LabelI=Iabc  Ipu=off  Pbase=100e6  Vbase=500e3  OutputType=Complex  PhasorSimulation=off  PSBequivalent=0
  genset  controller : Subsystem  mask{Vbase=208, Sbase=12500}
  a : PMIOPort  Port=1  Side=Right
  b : PMIOPort  Port=2  Side=Right
  c : PMIOPort  Port=3  Side=Right
  PQ : Outport  OutDataType=fixdt(1, 16)  OutScaling=2^0
  V : Outport  Port=2  OutDataType=fixdt(1, 16)  OutScaling=2^0
  I : Outport  Port=3  OutDataType=fixdt(1, 16)  OutScaling=2^0
  RMS : Outport  Port=4  OutDataType=fixdt(1, 16)  OutScaling=2^0
  freq : Outport  Port=5  OutDataType=fixdt(1, 16)  OutScaling=2^0
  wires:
  genset  controller/1(Pmech) -> Synchronous Machine pu Standard/1  "Pmec (pu)"
  genset  controller/2(Vf) -> Synchronous Machine pu Standard/2  "Vf (pu)"
  Synchronous Machine pu Standard/1 -> Bus Selector/1
  Bus Selector/1 -> genset  controller/1(wr)  "<Rotor speed  wm  (pu)>"
  Three-Phase V-I Measurement/1 -> genset  controller/2(Vabc), 3-phase  Instantaneous  Active & Reactive Power/1, RMS block2/1, V/1
  Three-Phase V-I Measurement/2 -> genset  controller/3(Iabc), 3-phase  Instantaneous  Active & Reactive Power/2, RMS block/1, I/1
  Preq/1 -> genset  controller/4(Preq)
  Ereq/1 -> genset  controller/5(Ereq1)
  genset  controller/3(w) -> Gain/1
  Gain/1 -> freq/1
  3-phase  Instantaneous  Active & Reactive Power/1 -> PQ/1
  RMS block2/1 -> Mux/1
  RMS block/1 -> Mux/2
  Mux/1 -> RMS/1
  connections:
  Three-Phase Series RLC Branch/RConn2 -- Three-Phase Series RLC Branch/RConn1 -- Ground/LConn1 -- Three-Phase Series RLC Branch/RConn3
  Synchronous Machine pu Standard/RConn1 -- T1/LConn1 -- Three-Phase Series RLC Branch/LConn1
  Synchronous Machine pu Standard/RConn2 -- T1/LConn2 -- Three-Phase Series RLC Branch/LConn2
  Synchronous Machine pu Standard/RConn3 -- T1/LConn3 -- Three-Phase Series RLC Branch/LConn3
  T1/RConn2 -- Three-Phase V-I Measurement/LConn2
  T1/RConn1 -- Three-Phase V-I Measurement/LConn1
  T1/RConn3 -- Three-Phase V-I Measurement/LConn3
  Three-Phase V-I Measurement/RConn1 -- a/RConn1
  b/RConn1 -- Three-Phase V-I Measurement/RConn2
  c/RConn1 -- Three-Phase V-I Measurement/RConn3
